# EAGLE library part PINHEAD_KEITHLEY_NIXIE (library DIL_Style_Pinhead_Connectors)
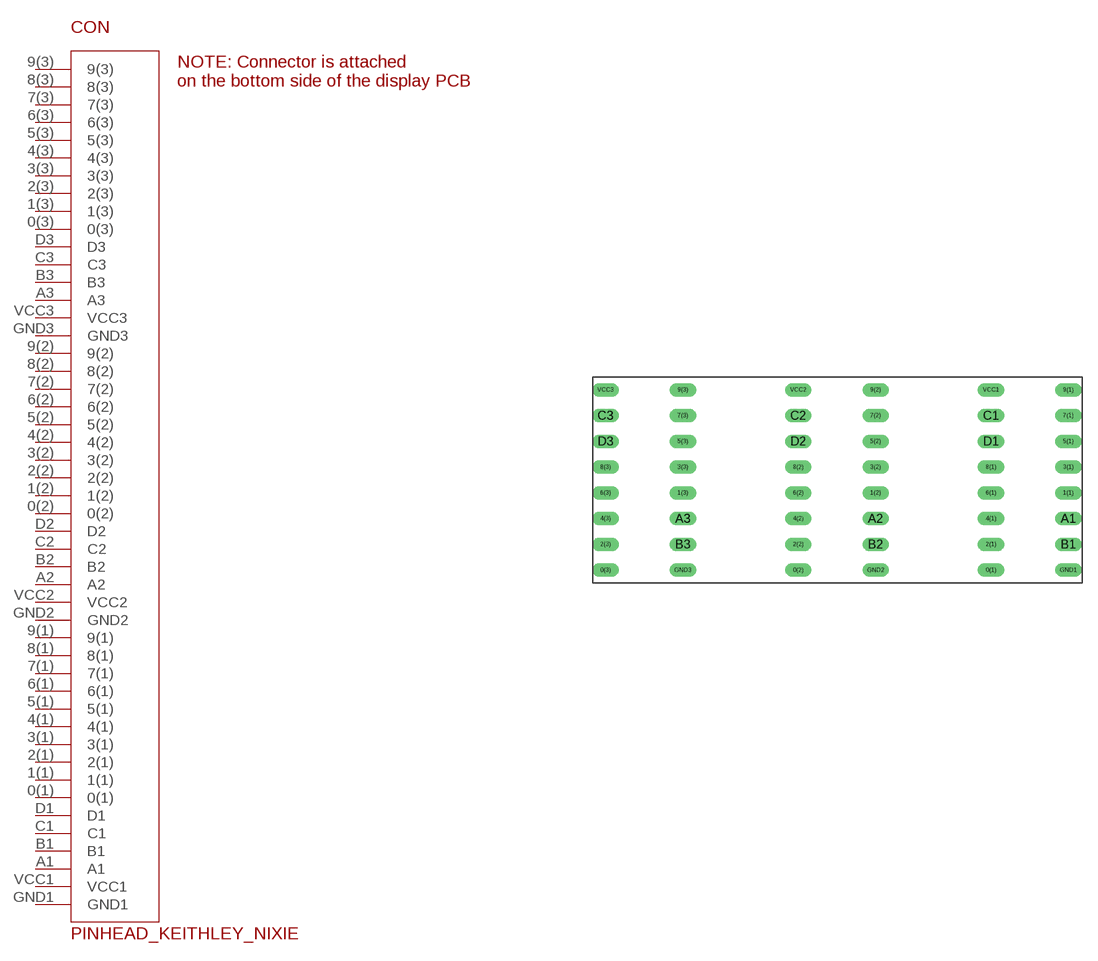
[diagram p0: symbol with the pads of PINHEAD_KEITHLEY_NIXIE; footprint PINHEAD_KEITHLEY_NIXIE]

Designator prefix CON

## PINHEAD_KEITHLEY_NIXIE  [PINHEAD_KEITHLEY_NIXIE]
0(1)  0(1)
0(2)  0(2)
0(3)  0(3)
1(1)  1(1)
1(2)  1(2)
1(3)  1(3)
2(1)  2(1)
2(2)  2(2)
2(3)  2(3)
3(1)  3(1)
3(2)  3(2)
3(3)  3(3)
4(1)  4(1)
4(2)  4(2)
4(3)  4(3)
5(1)  5(1)
5(2)  5(2)
5(3)  5(3)
6(1)  6(1)
6(2)  6(2)
6(3)  6(3)
7(1)  7(1)
7(2)  7(2)
7(3)  7(3)
8(1)  8(1)
8(2)  8(2)
8(3)  8(3)
9(1)  9(1)
9(2)  9(2)
9(3)  9(3)
A1  A1
A2  A2
A3  A3
B1  B1
B2  B2
B3  B3
C1  C1
C2  C2
C3  C3
D1  D1
D2  D2
D3  D3
GND1  GND1
GND2  GND2
GND3  GND3
VCC1  VCC1
VCC2  VCC2
VCC3  VCC3

## Footprint PINHEAD_KEITHLEY_NIXIE (pad centres in mm)
drill 0.8 long: 0(1) 38,-17.78; 0(2) 19,-17.78; 0(3) 0,-17.78; 1(1) 45.62,-10.16; 1(2) 26.62,-10.16; 1(3) 7.62,-10.16; 2(1) 38,-15.24; 2(2) 19,-15.24; 2(3) 0,-15.24; 3(1) 45.62,-7.62; 3(2) 26.62,-7.62; 3(3) 7.62,-7.62; 4(1) 38,-12.7; 4(2) 19,-12.7; 4(3) 0,-12.7; 5(1) 45.62,-5.08; 5(2) 26.62,-5.08; 5(3) 7.62,-5.08; 6(1) 38,-10.16; 6(2) 19,-10.16; 6(3) 0,-10.16; 7(1) 45.62,-2.54; 7(2) 26.62,-2.54; 7(3) 7.62,-2.54; 8(1) 38,-7.62; 8(2) 19,-7.62; 8(3) 0,-7.62; 9(1) 45.62,0; 9(2) 26.62,0; 9(3) 7.62,0; A1 45.62,-12.7; A2 26.62,-12.7; A3 7.62,-12.7; B1 45.62,-15.24; B2 26.62,-15.24; B3 7.62,-15.24; C1 38,-2.54; C2 19,-2.54; C3 0,-2.54; D1 38,-5.08; D2 19,-5.08; D3 0,-5.08; GND1 45.62,-17.78; GND2 26.62,-17.78; GND3 7.62,-17.78; VCC1 38,0; VCC2 19,0; VCC3 0,0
